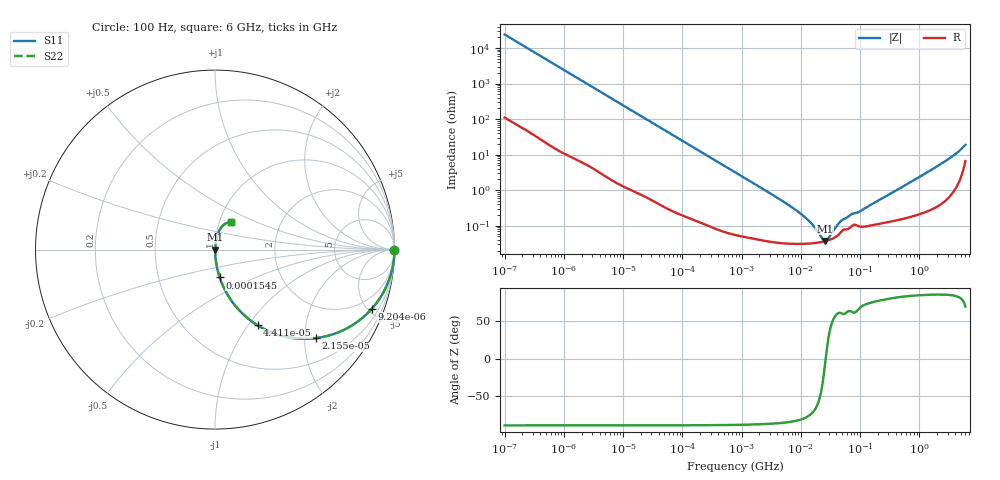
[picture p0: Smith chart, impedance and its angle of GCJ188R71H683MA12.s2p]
!Murata Part Number: GCJ188R71H683MA12
!These Parameters are Measured in Series Mode Connection
!Data Generated on Mar 13, 2026
!  o--ll--o
!Port1  Port2
!  o------o
!Operation Temp=25[degC], DC Bias Voltage=0[V]
!Freq. Start=100[Hz] Stop=6[GHz] 401[Steps]
# Hz S RI R 50
!Freq.(Hz) S11(Real) S11(Imag) S21(Real) S21(Imag) S12(Real) S12(Imag) S22(Real) S22(Imag)
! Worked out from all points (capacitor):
!   401 points, 100 Hz to 6 GHz, reference 50 ohm
!   read as one part in series: C = 66.1 nF near 109 Hz
!   lowest |Z| = 37.1 mohm at 25.46 MHz (marker M1)
!   series resonance near 26.31 MHz, so ESL is about 550 pH
!   S11 on the Smith chart (normalised r, x): 100 Hz: open; 9.204 kHz: 1.03, -5.29; 21.55 kHz: 1.01, -2.27; 44.11 kHz: 1.01, -1.11; 154.5 kHz: 1.00, -0.32; 6 GHz: 1.13, +0.35
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100  1 -0.00416  3.64e-05 0.00416  3.64e-05 0.00416  1 -0.00416
2008  0.9928 -0.0822  0.00723 0.0822  0.00723 0.0822  0.9928 -0.0822
4918  0.9598 -0.1939  0.0402 0.1939  0.0402 0.1939  0.9598 -0.1939
9204  0.8737 -0.3296  0.1263 0.3296  0.1263 0.3296  0.8737 -0.3296
13772  0.7569 -0.4262  0.2431 0.4262  0.2431 0.4262  0.7569 -0.4262
21550  0.5619 -0.4931  0.4381 0.4931  0.4381 0.4931  0.5619 -0.4931
40335  0.2707 -0.441  0.7293 0.441  0.7293 0.441  0.2707 -0.441
44113  0.2372 -0.422  0.7628 0.422  0.7628 0.422  0.2372 -0.422
75495  0.0973 -0.2928  0.9027 0.2928  0.9027 0.2928  0.0973 -0.2928
154540  0.0261 -0.1549  0.9739 0.1549  0.9739 0.1549  0.0261 -0.1549
774597  0.00157 -0.0319  0.9984 0.0319  0.9984 0.0319  0.00157 -0.0319
6644369  0.000323 -0.00354  0.9997 0.00354  0.9997 0.00354  0.000323 -0.00354
1.087309e7  0.000313 -0.00192  0.9997 0.00192  0.9997 0.00192  0.000313 -0.00192
1.555665e7  0.000321 -0.00105  0.9997 0.00105  0.9997 0.00105  0.000321 -0.00105
2.327686e7  0.000353 -0.000234  0.9996 0.000234  0.9996 0.000234  0.000353 -0.000234
2.545746e7  0.000366 -6.28e-05  0.9996 6.28e-05  0.9996 6.28e-05  0.000366 -6.28e-05
2.911731e7  0.00039 0.000194  0.9996 -0.000194  0.9996 -0.000194  0.00039 0.000194
3.983537e7  0.000497 0.000821  0.9995 -0.000821  0.9995 -0.000821  0.000497 0.000821
4.983056e7  0.000719 0.00125  0.9993 -0.00125  0.9993 -0.00125  0.000719 0.00125
3.124326e8  0.00134 0.00754  0.9987 -0.00754  0.9987 -0.00754  0.00134 0.00754
2.34314e9  0.00706 0.0546  0.9929 -0.0546  0.9929 -0.0546  0.00706 0.0546
6e9  0.087 0.1519  0.913 -0.1519  0.913 -0.1519  0.087 0.1519
